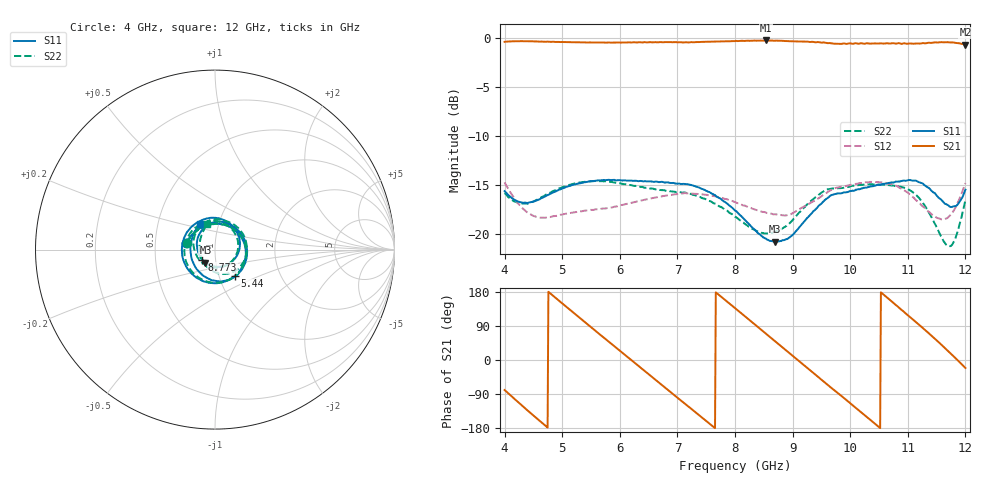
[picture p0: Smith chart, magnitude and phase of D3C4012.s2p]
! 11/4/2020 8:37:57 AM
! C:\USERS\KOBYR\DESKTOP\4.0 - 12.0 GHZ (D3I4012).S2P
! CHANNEL.1
! TR.MEASUREMENT
! CORRECTED.DATA
# GHZ S RI R 50.0
! FREQ.GHZ  S11RE  S11IM  S21RE  S21IM  S12RE  S12IM  S22RE  S22IM
!; PortSelection: Port_12
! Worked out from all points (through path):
!   601 points, 4 GHz to 12 GHz, reference 50 ohm
!   highest |S21| = -0.26 dB at 8.533 GHz (marker M1); lowest = -0.7 dB at 12 GHz (marker M2)
!   lowest |S11| = -20.8 dB at 8.693 GHz (marker M3), VSWR 1.20, Z = 44.5 - j6.6 ohm
!   |S11| at or under -10 dB: start of sweep to end of sweep
!   |S22| runs from -21.3 to -14.6 dB; largest |S21 - S12| = 0.96
!   S11 on the Smith chart (normalised r, x): 4 GHz: 0.72, +0.06; 5.44 GHz: 1.19, -0.36; 8.773 GHz: 0.86, -0.10; 12 GHz: 0.81, +0.24
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4  -0.16 0.0391  0.1781 -0.9379  -0.1768 -0.0457  -0.1564 0.0385
4.306667  -0.0513 0.1342  -0.4935 -0.8258  -0.1317 0.0294  -0.0489 0.1337
4.693333  0.1053 0.1126  -0.9447 -0.1423  -0.0901 0.0798  0.1069 0.1136
4.986667  0.1685 0.0151  -0.8341 0.4608  -0.0458 0.1161  0.1708 0.0173
5.346667  0.1358 -0.1211  -0.2584 0.9123  0.0354 0.1251  0.141 -0.1168
5.44  0.1098 -0.1477  -0.0685 0.9452  0.0571 0.1178  0.1161 -0.1435
6.093333  -0.1314 -0.133  0.9232 0.213  0.1401 -0.0178  -0.1172 -0.135
6.666667  -0.1678 0.0743  0.5038 -0.8051  0.0407 -0.1481  -0.1572 0.06
7.04  -0.0693 0.1659  -0.234 -0.9213  -0.0822 -0.1374  -0.0659 0.1488
7.453333  0.0758 0.15  -0.8649 -0.4013  -0.1574 -0.0173  0.0713 0.1331
8  0.1302 -0.0162  -0.7032 0.6576  -0.0685 0.1275  0.1188 -0.0268
8.533333  -0.00776 -0.094  0.3314 0.9119  0.0663 0.1096  -0.0237 -0.0971
8.693333  -0.0532 -0.0735  0.6234 0.7395  0.0923 0.0849  -0.0699 -0.0743
8.773333  -0.0717 -0.0566  0.743 0.6174  0.1023 0.0705  -0.0879 -0.0562
9.346667  -0.0768 0.1028  0.8056 -0.5124  0.1323 -0.0598  -0.0906 0.1184
9.946667  0.0938 0.1329  -0.2748 -0.8911  -0.0393 -0.1714  0.0868 0.1492
10.33333  0.164 0.0567  -0.8546 -0.3798  -0.1677 -0.0741  0.1607 0.0774
10.66667  0.1777 -0.0363  -0.8872 0.3002  -0.1643 0.0722  0.1764 -0.0104
11.01333  0.1264 -0.1384  -0.4194 0.8355  -0.0472 0.1534  0.131 -0.1049
11.32  0.00196 -0.1742  0.2181 0.9136  0.0439 0.125  0.0229 -0.1331
11.69333  -0.13 -0.0516  0.8643 0.396  0.087 0.0833  -0.0828 -0.0248
12  -0.086 0.1437  0.8627 -0.3325  0.1699 0.0627  -0.0435 0.1414
